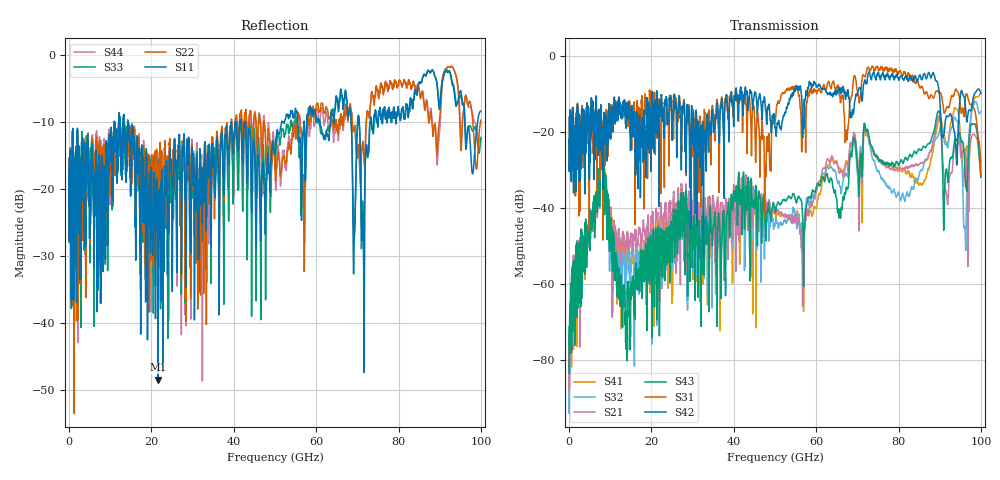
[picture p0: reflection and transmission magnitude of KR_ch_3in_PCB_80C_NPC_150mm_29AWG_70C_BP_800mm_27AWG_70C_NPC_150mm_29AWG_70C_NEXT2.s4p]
# GHz S RI R 45
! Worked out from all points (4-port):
!   4000 points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, 25 MHz to 100 GHz, reference 45 ohm
!   strongest paths, dB at 25 MHz, 25.02 GHz, 50.02 GHz, 75.03 GHz, 100 GHz:
!     S42: -21.8, -20.6, -18.8, -4.2, -9.7
!     S31: -21.7, -16.7, -16.6, -3.1, -31.3
!     S43: -83.3, -51.2, -40.5, -26.4, -31.8
!     S21: -81.0, -46.8, -40.4, -27.2, -27.3
!     S32: -83.1, -50.8, -44.7, -30.4, -14.5
!     S41: -88.0, -65.0, -41.2, -27.1, -9.7
!   lowest |S11| = -48.4 dB at 21.6 GHz (marker M1), VSWR 1.01, Z = 44.7 - j0.165 ohm
!   |S11| at or under -10 dB: start of sweep to 11 GHz; 14.35 GHz to 39.33 GHz (24.98 GHz wide, 93.1 % of centre); 42.86 GHz to 51.61 GHz (8.748 GHz wide, 18.5 % of centre)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
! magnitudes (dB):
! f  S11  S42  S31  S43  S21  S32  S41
! 25 MHz  -17.2  -21.8  -21.7  -83.3  -81.0  -83.1  -88.0
! 8.025 GHz  -16.4  -26.0  -22.9  -25.7  -26.4  -26.4  -26.0
! 13.65 GHz  -12.9  -15.0  -14.1  -70.6  -50.5  -58.5  -53.8
! 21.6 GHz  -48.4  -14.4  -20.0  -45.9  -43.5  -46.6  -44.5
! 71.95 GHz  -15.3  -6.5  -5.3  -18.9  -19.4  -18.7  -20.0
! 96.1 GHz  -9.6  -11.6  -13.3  -28.6  -24.7  -44.8  -27.3
! 100 GHz  -8.3  -9.7  -31.3  -31.8  -27.3  -14.5  -9.7
